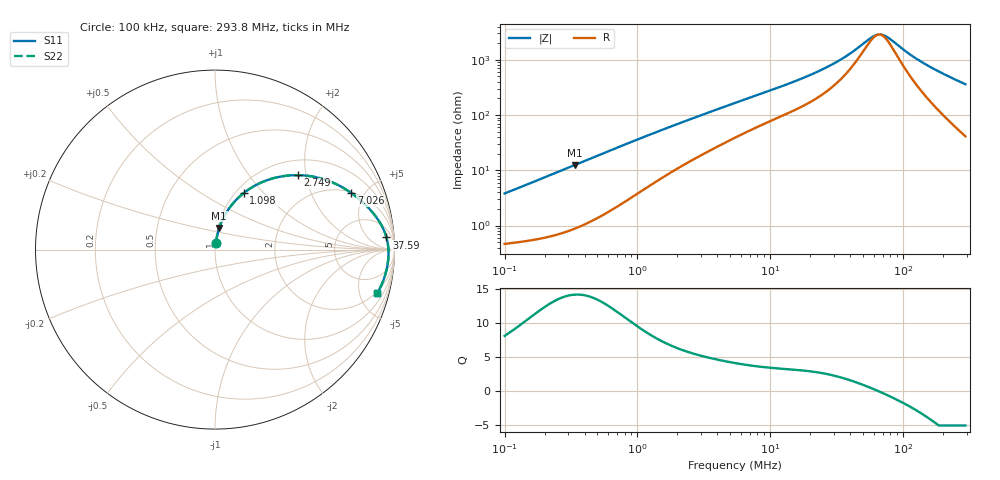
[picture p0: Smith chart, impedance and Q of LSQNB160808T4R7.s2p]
! LSQNB160808T4R7  S-PARAMETER MODEL  ( General Type )
! Model Generated by TAIYO YUDEN Corporation (http://www.ty-top.com)
! Version 2.0
! TAIYO YUDEN Control No. 100810NF25SB-FKC
! Copyright(c) 2007 TAIYO YUDEN CO.,LTD. All Rights Reserved.
! Product Description (link to TY-COMPAS)
! https://ds.yuden.co.jp/TYCOMPAS/or/detail?pn=LSQNB160808T4R7M&u=M
! Products Name : Inductors
! Characteristics :
!  Inductance : 4.7 uH , SRF(min) : 45 MHz , DC Resistance(max) : 0.312 Ohm
!  Rated Current : Saturation :145 mA , Temp Rise : 470 mA (40 degC)
!  Case Size : 1.6 x 0.8 / 0.063 x 0.031 [mm/inch] , Thickness : 0.8 / 0.031 [mm/inch]
!  (Conditions: Temperature = 25 degC , DC Bias Current/Voltage = 0A / 0V)
! External Node Assignments :
!  1  o---GGG---o  2
! GND o---------o GND
! Frequency Range : 0.1MHz  -  293.796821MHz  [ 402 STEP ]
# MHz S RI R 50
! Freq[MHz].  S11 Real  S11 Imag  S21 Real  S21 Imag  S12 Real  S12 Imag  S22 Real  S22 Imag
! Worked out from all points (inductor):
!   401 points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, 100 kHz to 293.8 MHz, reference 50 ohm
!   read as one part in series: L = 5.96 uH near 104.1 kHz
!   highest Q = 14.2 at 338 kHz (marker M1), where L = 5.87 uH
!   self-resonance near 65.59 MHz
!   S11 on the Smith chart (normalised r, x): 100 kHz: 1.01, +0.08; 1.098 MHz: 1.09, +0.78; 2.749 MHz: 1.33, +1.80; 7.026 MHz: 2.05, +4.00; 37.59 MHz: 13, +21; 293.8 MHz: 1.82, -7.17
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0.1  0.00603 0.0373  0.994 -0.0373  0.994 -0.0373  0.00603 0.0373
0.337969  0.0236 0.1206  0.9764 -0.1206  0.9764 -0.1206  0.0236 0.1206
0.380976  0.0286 0.1349  0.9714 -0.1349  0.9714 -0.1349  0.0286 0.1349
0.679722  0.0749 0.2244  0.9251 -0.2244  0.9251 -0.2244  0.0749 0.2244
1.097524  0.1603 0.3154  0.8397 -0.3154  0.8397 -0.3154  0.1603 0.3154
1.451429  0.2364 0.3638  0.7636 -0.3638  0.7636 -0.3638  0.2364 0.3638
2.037923  0.3511 0.404  0.6489 -0.404  0.6489 -0.404  0.3511 0.404
2.74941  0.4629 0.4148  0.5371 -0.4148  0.5371 -0.4148  0.4629 0.4148
5.420303  0.6932 0.356  0.3068 -0.356  0.3068 -0.356  0.6932 0.356
7.026436  0.759 0.3158  0.241 -0.3158  0.241 -0.3158  0.759 0.3158
13.04694  0.869 0.2174  0.131 -0.2174  0.131 -0.2174  0.869 0.2174
20.65007  0.92 0.149  0.08 -0.149  0.08 -0.149  0.92 0.149
28.42126  0.9427 0.1043  0.0573 -0.1043  0.0573 -0.1043  0.9427 0.1043
37.5859  0.9554 0.0677  0.0446 -0.0677  0.0446 -0.0677  0.9554 0.0677
56.03086  0.9648 0.0188  0.0352 -0.0188  0.0352 -0.0188  0.9648 0.0188
61.91244  0.9659 0.0069  0.0341 -0.0069  0.0341 -0.0069  0.9659 0.0069
69.79087  0.9667 -0.00745  0.0333 0.00745  0.0333 0.00745  0.9667 -0.00745
78.67184  0.9669 -0.022  0.0331 0.022  0.0331 0.022  0.9669 -0.022
108.2782  0.9643 -0.0629  0.0357 0.0629  0.0357 0.0629  0.9643 -0.0629
140.363  0.9584 -0.1003  0.0416 0.1003  0.0416 0.1003  0.9584 -0.1003
201.055  0.9415 -0.1615  0.0585 0.1615  0.0585 0.1615  0.9415 -0.1615
293.7968  0.905 -0.2414  0.095 0.2414  0.095 0.2414  0.905 -0.2414
